PROGRAM LIVINGROOM
VAR	
	fbLight1: FB_Light;
	fbLight2: FB_Light;
	fbLight3: FB_Light;
	
	R_TRIG_BlindUp1: R_TRIG;	
	R_TRIG_BlindDown1: R_TRIG;
	bSwitchBlindUp1: BOOL;
	bSwitchBlindDown1: BOOL;
	fbVenetianBlind1: FB_VenetianBlind;	
	
	R_TRIG_BlindUp2: R_TRIG;	
	R_TRIG_BlindDown2: R_TRIG;
	bSwitchBlindUp2: BOOL;
	bSwitchBlindDown2: BOOL;
	fbVenetianBlind2: FB_VenetianBlind;	
END_VAR
VAR_OUTPUT
	rTemperature: LREAL;
END_VAR

// Light 1
fbLight1(bOn:= , bOff:= , bToggle:= GVL.I_bTerm1_Var10, bLight=> GVL.Q_bTerm3_Var8);

// Light 2
fbLight2(bOn:= , bOff:= , bToggle:= GVL.I_bTerm1_Var11, bLight=> GVL.Q_bTerm3_Var9);
	
// Light 3
fbLight3(bOn:= , bOff:= , bToggle:= GVL.I_bTerm1_Var12, bLight=> GVL.Q_bTerm3_Var10);

	
// Blind 1
R_TRIG_BlindUp1(CLK:=GVL.I_bTerm1_Var13);
bSwitchBlindUp1:=R_TRIG_BlindUp1.Q;
R_TRIG_BlindDown1(CLK:=GVL.I_bTerm1_Var14);
bSwitchBlindDown1:= R_TRIG_BlindDown1.Q;

fbVenetianBlind1(
	bUp:= bSwitchBlindUp1, 
	bDown:= bSwitchBlindDown1, 
	bStop:= (bSwitchBlindUp1 OR bSwitchBlindDown1) AND (fbVenetianBlind1.bBlindUp OR fbVenetianBlind1.bBlindDown), 
	bSwitchOverUp:= , 
	bSwitchOverDown:= , 
	tSwitchOverTime:= , 
	bStepUp:= , 
	bStepDown:= , 
	tStepTime:= , 
	bShadowPosition:= , 
	tShadowTurnAroundTime:= , 
	tShadowTurnOffTime:= , 
	bSafetyPosition:= , 
	tTurnOffTime:= , 
	tSwitchOverDeadTime:= , 
	bBlindUp=> GVL.Q_bTerm7_Var1, 
	bBlindDown=> GVL.Q_bTerm7_Var2);
	
// Blind 2
R_TRIG_BlindUp2(CLK:=GVL.I_bTerm1_Var15);
bSwitchBlindUp2:=R_TRIG_BlindUp2.Q;
R_TRIG_BlindDown2(CLK:=GVL.I_bTerm1_Var16);
bSwitchBlindDown2:= R_TRIG_BlindDown2.Q;

fbVenetianBlind2(
	bUp:= bSwitchBlindUp2, 
	bDown:= bSwitchBlindDown2, 
	bStop:= (bSwitchBlindUp2 OR bSwitchBlindDown2) AND (fbVenetianBlind2.bBlindUp OR fbVenetianBlind2.bBlindDown), 
	bSwitchOverUp:= , 
	bSwitchOverDown:= , 
	tSwitchOverTime:= , 
	bStepUp:= , 
	bStepDown:= , 
	tStepTime:= , 
	bShadowPosition:= , 
	tShadowTurnAroundTime:= , 
	tShadowTurnOffTime:= , 
	bSafetyPosition:= , 
	tTurnOffTime:= , 
	tSwitchOverDeadTime:= , 
	bBlindUp=> GVL.Q_bTerm8_Var1, 
	bBlindDown=> GVL.Q_bTerm8_Var2);
	
// Temperature
rTemperature := INT_TO_LREAL(GVL.I_nTerm5_Var2) / 10;

END_PROGRAM
